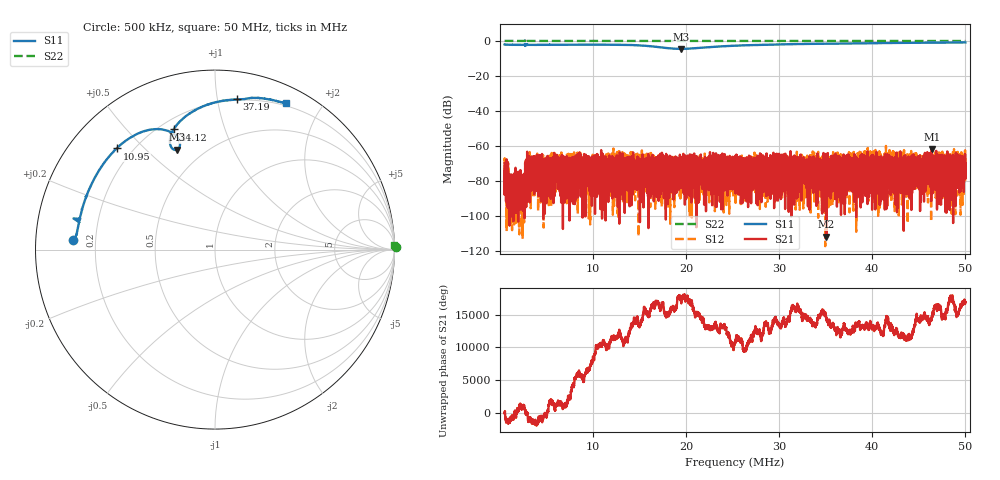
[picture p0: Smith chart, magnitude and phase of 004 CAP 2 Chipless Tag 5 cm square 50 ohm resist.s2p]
!  26/06/2025  15:21:55
! Ref Plane: 0.000 mm
# MHZ S MA R  50
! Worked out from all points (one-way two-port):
!   10001 points, 500 kHz to 50 MHz, reference 50 ohm
!   highest |S21| = -61.80 dB at 46.41 MHz (marker M1); lowest = -111.6 dB at 35.07 MHz (marker M2)
!   lowest |S11| = -4.5 dB at 19.42 MHz (marker M3), VSWR 3.94, Z = 18.2 + j31.3 ohm
!   |S11| at or under -10 dB: nowhere
!   |S22| runs from -0.3 to 0.3 dB; largest |S21 - S12| = 0.0013
!   S11 on the Smith chart (normalised r, x): 500 kHz: 0.12, +0.03; 10.95 MHz: 0.14, +0.42; 24.12 MHz: 0.25, +0.68; 37.19 MHz: 0.19, +1.14; 50 MHz: 0.17, +1.58
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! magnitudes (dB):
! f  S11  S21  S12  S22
! 500 kHz  -2.0  -69.7  -77.3  0.1
! 1.054 MHz  -2.2  -85.8  -90.5  0.0
! 1.599 MHz  -2.2  -92.3  -89.5  0.0
! 2.45 MHz  -2.2  -82.8  -91.8  0.0
! 3.03 MHz  -2.2  -91.5  -72.8  0.0
! 8.752 MHz  -2.1  -79.9  -75.4  0.0
! 10.95 MHz  -2.1  -73.1  -79.0  0.0
! 17 MHz  -3.5  -65.4  -78.2  0.0
! 19.42 MHz  -4.5  -68.5  -71.4  0.0
! 24.12 MHz  -3.0  -85.3  -77.8  0.0
! 25.25 MHz  -2.7  -72.3  -76.2  0.0
! 33.5 MHz  -1.7  -75.0  -73.6  0.0
! 35.07 MHz  -1.6  -111.6  -64.6  0.0
! 37.19 MHz  -1.5  -71.3  -73.3  0.0
! 39.29 MHz  -1.4  -71.9  -75.1  0.0
! 41.04 MHz  -1.2  -77.0  -73.5  0.0
! 41.75 MHz  -1.2  -66.2  -70.0  0.0
! 46.41 MHz  -1.0  -61.8  -65.6  0.0
! 48.03 MHz  -0.9  -75.1  -73.7  0.0
! 48.72 MHz  -0.9  -65.6  -66.7  0.0
! 49.73 MHz  -0.9  -69.9  -67.0  0.0
! 50 MHz  -0.9  -70.0  -75.6  0.0
